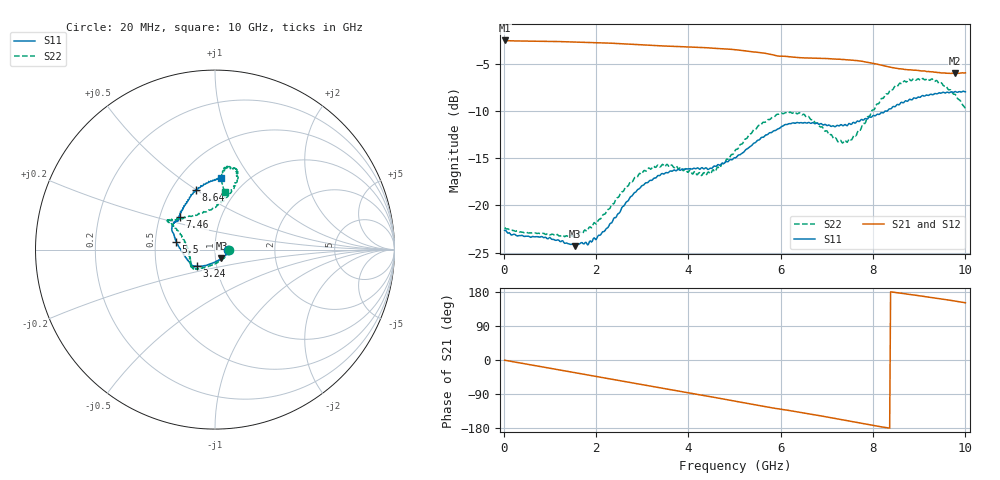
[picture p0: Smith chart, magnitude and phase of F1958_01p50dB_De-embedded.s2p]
! Integrated Device Technology
! Corporate Headquarters
! 6024 Silver Creek Valley Road
! San Jose, CA 95138  USA
! Phone:  1-408-284-8200
! Toll Free:  1-800-223-1366
! Webpage:  http://www.idt.com/
! Timing and RF Division
! 515 Groton Road, Suite 102
! Westford, MA 01886-6024
! Device:  F1958
! Description: 7-bit 0.25 dB Digital Step Attenuator
! Frequency:  0.001 -  6.000 GHz
! Package:  4x4 mm Thin QFN Plastic Package: 24 pin
! Ports:  2 RF, 12 DC
!  Pin  1  = D0
!  Pin  2  = VDD
!  Pin  3  = VMODE
!  Pin  4  = GND
!  Pin  5  = RF1  =  Port 1
!  Pin  6  = GND
!  Pin  7  = GND
!  Pin  8  = GND
!  Pin  9  = GND
!  Pin 10  = GND
!  Pin 11  = GND
!  Pin 12  = GND
!  Pin 13  = GND
!  Pin 14  = RF2  =  Port 2
!  Pin 15  = GND
!  Pin 16  = LE
!  Pin 17  = CLK
!  Pin 18  = DATA
!  Pin 19  = D6
!  Pin 20  = D5
!  Pin 21  = D4
!  Pin 22  = D3
!  Pin 23  = D2
!  Pin 24  = D1
! State:  6
! Atten State:  1.50 dB
! Voltage:  +3.30 Volts
! Current:  0.257 mA
! Data:  The device was measured on a F1958 evaluation board which has
!  individual transmission lines to the RF pins.  Data was collected
!  using a calibrated network analyzer.  The evaluation board was
!  de-embedded using Automatic Fixture Removal (AFR).
!  The reference plane is the edge of the package pin.
! Misc:
!  Action Tracker AT0419
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# GHz S dB R 50
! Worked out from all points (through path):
!   500 points, 20 MHz to 10 GHz, reference 50 ohm
!   highest |S21| = -2.54 dB at 20 MHz (marker M1); lowest = -6.0 dB at 9.78 GHz (marker M2)
!   group delay of S21, straight-line fit = 58.8 ps
!   lowest |S11| = -24.3 dB at 1.54 GHz (marker M3), VSWR 1.13, Z = 53.5 - j5.25 ohm
!   |S11| at or under -10 dB: start of sweep to 8.31 GHz
!   |S22| runs from -23.3 to -6.6 dB; largest |S21 - S12| = 0.0022
!   S11 on the Smith chart (normalised r, x): 20 MHz: 1.16, -0.01; 3.24 GHz: 0.80, -0.15; 5.5 GHz: 0.64, +0.06; 7.46 GHz: 0.63, +0.25; 8.64 GHz: 0.66, +0.50; 10 GHz: 0.77, +0.73
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0.02  -22.65 -1.9  -2.54 -0.6  -2.54 -0.6  -22.35 -2.2
0.8  -23.34 -19.0  -2.63 -17.4  -2.63 -17.4  -23.01 -24.8
1.54  -24.33 -53.5  -2.70 -33.4  -2.70 -33.4  -23.11 -64.8
1.7  -23.96 -63.5  -2.73 -36.8  -2.72 -36.8  -23.00 -74.9
2.04  -23.26 -87.2  -2.78 -44.2  -2.77 -44.2  -21.67 -96.1
2.78  -19.01 -126.0  -2.94 -60.4  -2.93 -60.4  -17.51 -127.7
3.24  -17.19 -137.6  -3.08 -70.3  -3.07 -70.4  -15.85 -138.4
3.36  -16.85 -138.8  -3.10 -72.8  -3.11 -72.9  -15.82 -139.6
4.42  -16.20 -152.6  -3.32 -95.6  -3.33 -95.6  -16.51 -174.7
5.02  -14.96 -173.1  -3.52 -108.8  -3.53 -108.8  -14.13 159.1
5.5  -13.12 168.8  -3.80 -119.3  -3.81 -119.3  -11.65 150.2
6  -11.74 157.0  -4.20 -129.5  -4.22 -129.5  -10.23 148.7
6.4  -11.28 149.4  -4.36 -137.7  -4.38 -137.6  -10.19 147.6
6.68  -11.26 145.8  -4.41 -143.3  -4.43 -143.2  -10.93 143.3
7.22  -11.53 141.4  -4.53 -155.1  -4.54 -155.0  -13.11 120.2
7.46  -11.45 137.4  -4.59 -160.5  -4.60 -160.4  -13.17 100.5
7.96  -10.67 126.8  -4.93 -172.1  -4.93 -172.1  -10.15 76.0
8.34  -9.83 116.1  -5.33 -179.4  -5.34 -179.5  -8.09 72.0
8.64  -9.13 107.6  -5.57 175.6  -5.58 175.6  -7.05 73.5
9.28  -8.28 91.4  -5.87 164.3  -5.88 164.3  -6.61 82.5
9.78  -7.95 85.6  -6.03 155.6  -6.06 155.6  -8.25 83.6
10  -7.97 85.1  -5.96 151.1  -6.00 151.2  -9.74 80.1
